(* Logix 5000 AddOnInstructionDefinition export NORD_ADC; software revision 24.02; part 2 of 3 *)
(* tags used below, declared in another part *)
   ParameterNumber : INT;
   ParameterIndex : SINT;
   ParameterSet : SINT;
   Done : BOOL;
   Busy : BOOL;
   ReadMsg : MESSAGE;   // Read Msg to Module
   ReadTrigger : BOOL;
   ReadValue : DINT;   // Read Value from message
   WriteMsg : MESSAGE;   // Write Msg to Module
   WriteTrigger : BOOL;
   WriteValue : DINT;
   Error : BOOL;
   VFD_NotPresent : BOOL;   // VFD not present in Localbus
   EthernetDisconnected : BOOL;   // Eth. cord to Module is disconnected
   Backup : NORD_ParameterBackup;   // Parameter Backup File
   CompletionPercent : DINT;   // Backup/Restore Complete Percentage
   GetID_InProcess : BOOL;
   BackupInProcess : BOOL;
   RestoreInProcess : BOOL;
   HasInternalPLC : BOOL;
   ErrorID : DINT;   // Message Error Code
   WriteValueMSG : DINT;
   Instance : INT;
   HasParamIndex : BOOL;   // Set Parameter has Indexes
   HasParamSets : BOOL;   // Set Parameter has Parameter Sets
   ReadErrorOS : BOOL;
   WriteErrorONS : BOOL;
   TrigONS1 : BOOL;
   ReadDoneOS : BOOL;
   WriteDoneONS : BOOL;
   MacAddr : SINT[6];   // MAC Address of CU/TU
   GetID_ReadTrigger : BOOL;
   BackupSM : INT;   // 0: Not Active 10: Reset indexes 20: Clear Old Backup 30: Reset Indexes 40: Prepare Read Msg 50: Read Trigger 60: Read Co
   Index : INT;
   DeviceID : STRING;   // Device ID of VFD
   RestoreSM : INT;   // 0: Not Active 10: Reset Indexes 15: # of Saved Param 20: Get RestoreParam 21: Prepare Read Msg 22: Read Trigger 23: Read
   Index1 : INT;   // Store Index: VFD
   IndexInst : INT;   // Instance Index
   RestoreParam : INT;   // Parameter Number to be Restored
   SavedParamsVFD : INT;
   BackupReadTrigger : BOOL;
   RestWriteTrig : BOOL;
   RestIndexONS : BOOL;
   RestReadTrig : BOOL;
   BackupLast : BOOL;   // Determines Backup/Restore Complete Percentage Calculation
   WriteSM : SINT;   // 0: Not Active 10: Write LEN=4 20: 1st WriteTrigger 30: Write Complete - 40: Write LEN=2 - 50: 2nd WriteTrigger 60: Write
   Class : INT;
   TrigONS2 : BOOL;
   NumOfParams : DINT;   // Number of parameters in the VFD
   WriteTriggerONS : BOOL;
   WriteTrigInternal : BOOL;   // 1st Attempt: LEN = 4 2nd Attempt: LEN = 2
   Write16Bit : BOOL;   // 0: Write LEN=4 1: Write LEN=2
   AOI_FirstScan : BOOL;   // First Scan of AOI
   Percent100ONS : BOOL;
   GetID_Done_ONS : BOOL;
   Index2 : INT;   // Store Index: CU/TU
   SavedParamsCTU : INT;
   RestoreCTU : BOOL;   // Restore CTU Parameters
   RestIndexONS2 : BOOL;
   CompPercentIndex : INT;
   StoreDevID : BOOL;
   StoreDevID_DN : BOOL;
   ResetIndexes : BOOL;
   ResetIndexDN : BOOL;
   GetRestParam : BOOL;   // Get Restore Parameter Logic
   GetRestParamDN : BOOL;   // Got Restore Param
   ResetMsgEr : BOOL;
   RestoreFailed : BOOL;   // All writes in restore failed
   RestoreFailedONS : BOOL;
   RestoreHasWrite : BOOL;
   RestoreHasWriteONS : BOOL;
(* NORD_ADC, continued *)

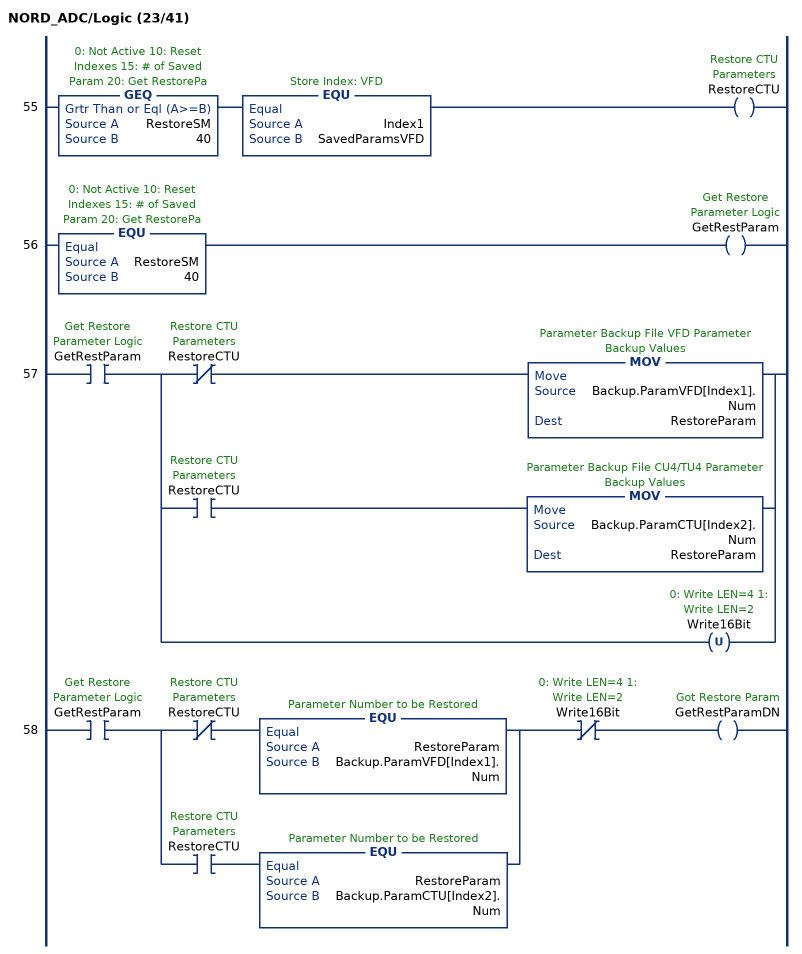
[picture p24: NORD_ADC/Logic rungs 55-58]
   55: GEQ(RestoreSM,40)EQU(Index1,SavedParamsVFD)OTE(RestoreCTU);
   56: EQU(RestoreSM,40)OTE(GetRestParam);
   57: XIC(GetRestParam)[XIO(RestoreCTU) MOV(Backup.ParamVFD[Index1].Num,RestoreParam) ,XIC(RestoreCTU) MOV(Backup.ParamCTU[Index2].Num,RestoreParam) ,OTU(Write16Bit) ];
   58: XIC(GetRestParam)[XIO(RestoreCTU) EQU(RestoreParam,Backup.ParamVFD[Index1].Num) ,XIC(RestoreCTU) EQU(RestoreParam,Backup.ParamCTU[Index2].Num) ]XIO(Write16Bit)OTE(GetRestParamDN);
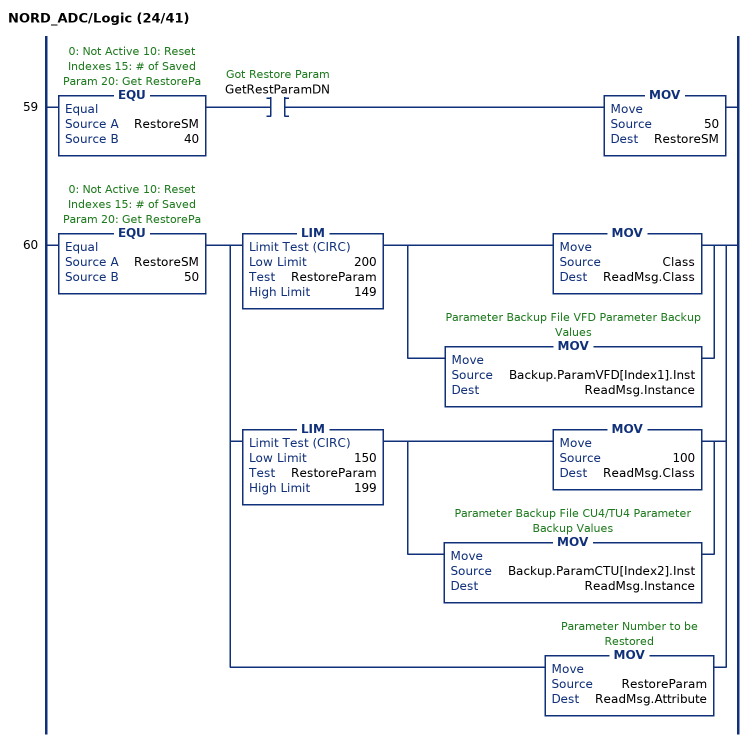
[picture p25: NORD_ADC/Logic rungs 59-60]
   59: EQU(RestoreSM,40)XIC(GetRestParamDN)MOV(50,RestoreSM);
   60: EQU(RestoreSM,50)[[LIM(200,RestoreParam,149) [MOV(Class,ReadMsg.Class) ,MOV(Backup.ParamVFD[Index1].Inst,ReadMsg.Instance) ] ,LIM(150,RestoreParam,199) [MOV(100,ReadMsg.Class) ,MOV(Backup.ParamCTU[Index2].Inst,ReadMsg.Instance) ] ] ,MOV(RestoreParam,ReadMsg.Attribute) ];
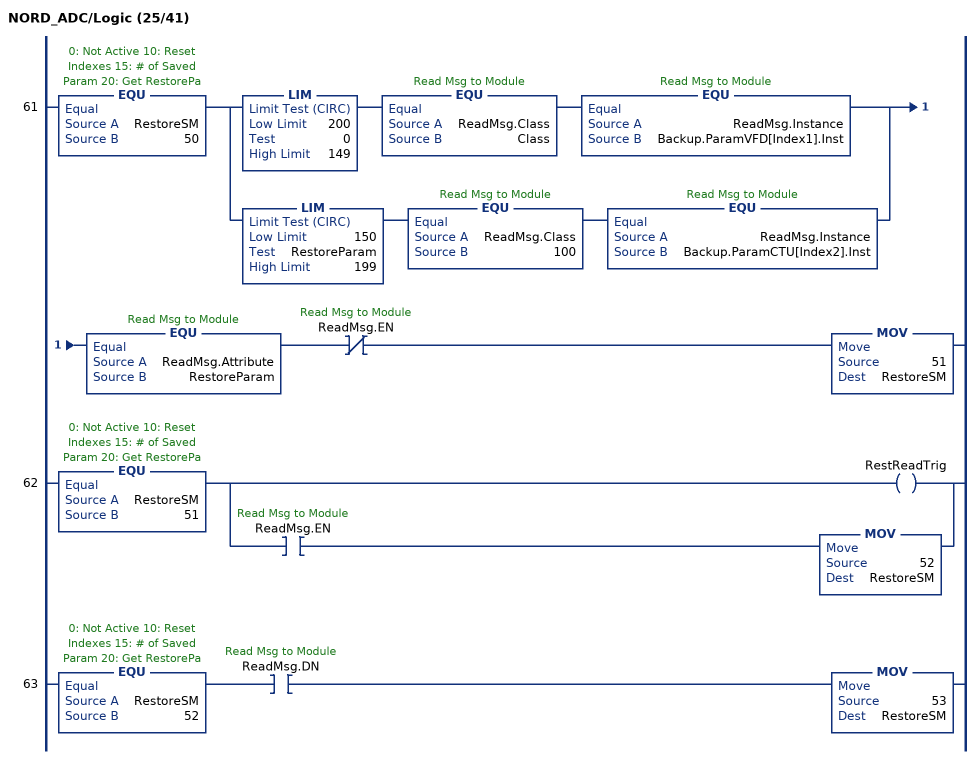
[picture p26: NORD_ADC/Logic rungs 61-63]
   61: EQU(RestoreSM,50)[LIM(200,0,149) EQU(ReadMsg.Class,Class) EQU(ReadMsg.Instance,Backup.ParamVFD[Index1].Inst) ,LIM(150,RestoreParam,199) EQU(ReadMsg.Class,100) EQU(ReadMsg.Instance,Backup.ParamCTU[Index2].Inst) ]EQU(ReadMsg.Attribute,RestoreParam)XIO(ReadMsg.EN)MOV(51,RestoreSM);
   62: EQU(RestoreSM,51)[OTE(RestReadTrig) ,XIC(ReadMsg.EN) MOV(52,RestoreSM) ];
   63: EQU(RestoreSM,52)XIC(ReadMsg.DN)MOV(53,RestoreSM);
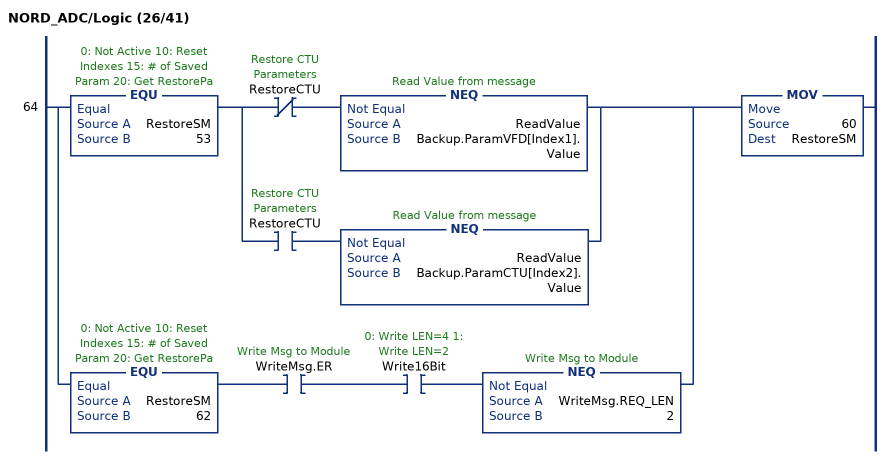
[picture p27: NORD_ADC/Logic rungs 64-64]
   64: [EQU(RestoreSM,53) [XIO(RestoreCTU) NEQ(ReadValue,Backup.ParamVFD[Index1].Value) ,XIC(RestoreCTU) NEQ(ReadValue,Backup.ParamCTU[Index2].Value) ] ,EQU(RestoreSM,62) XIC(WriteMsg.ER) XIC(Write16Bit) NEQ(WriteMsg.REQ_LEN,2) ]MOV(60,RestoreSM);
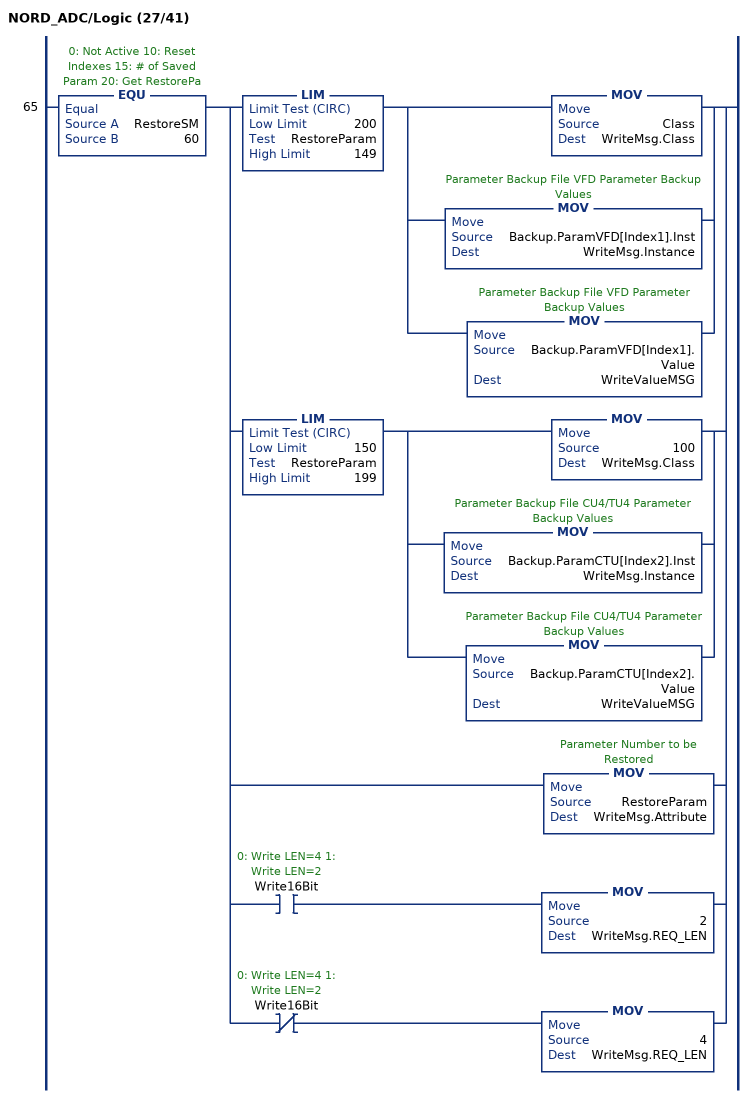
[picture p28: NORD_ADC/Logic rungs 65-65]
   65: EQU(RestoreSM,60)[[LIM(200,RestoreParam,149) [MOV(Class,WriteMsg.Class) ,[MOV(Backup.ParamVFD[Index1].Inst,WriteMsg.Instance) ,MOV(Backup.ParamVFD[Index1].Value,WriteValueMSG) ] ] ,LIM(150,RestoreParam,199) [MOV(100,WriteMsg.Class) ,MOV(Backup.ParamCTU[Index2].Inst,WriteMsg.Instance) ,MOV(Backup.ParamCTU[Index2].Value,WriteValueMSG) ] ] ,MOV(RestoreParam,WriteMsg.Attribute) ,XIC(Write16Bit) MOV(2,WriteMsg.REQ_LEN) ,XIO(Write16Bit) MOV(4,WriteMsg.REQ_LEN) ];
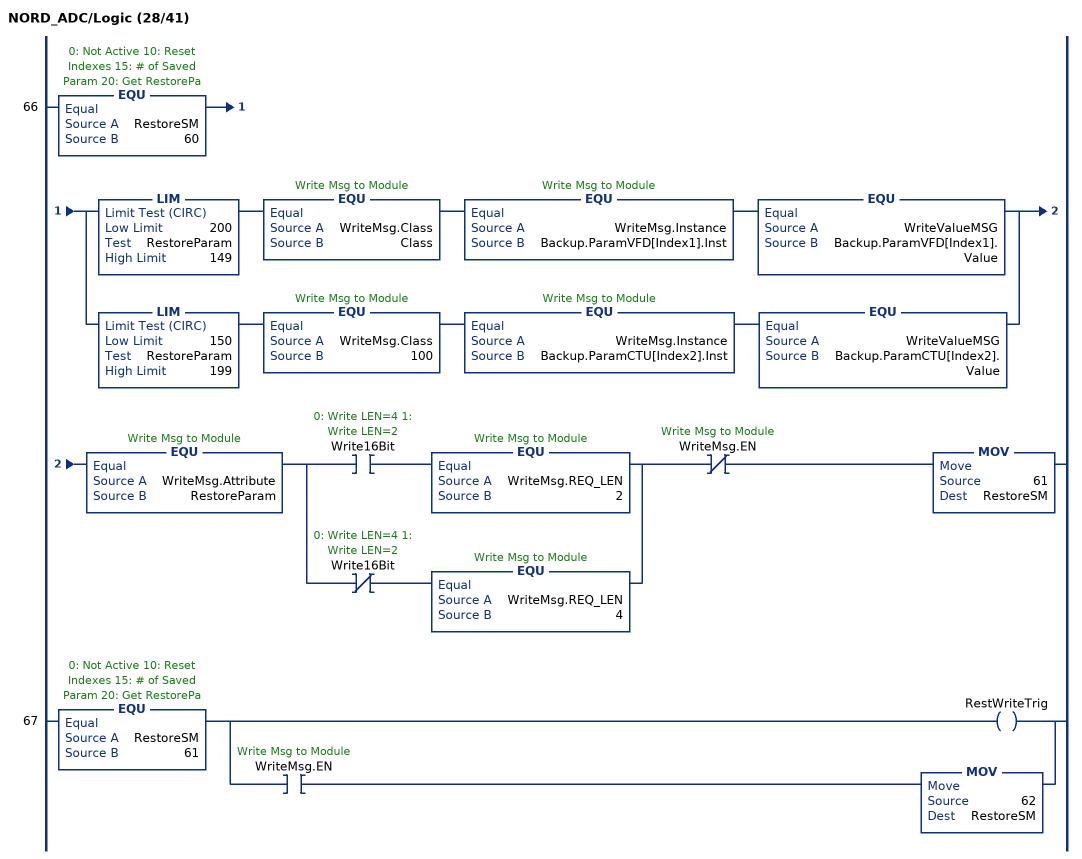
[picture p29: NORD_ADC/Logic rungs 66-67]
   66: EQU(RestoreSM,60)[LIM(200,RestoreParam,149) EQU(WriteMsg.Class,Class) EQU(WriteMsg.Instance,Backup.ParamVFD[Index1].Inst) EQU(WriteValueMSG,Backup.ParamVFD[Index1].Value) ,LIM(150,RestoreParam,199) EQU(WriteMsg.Class,100) EQU(WriteMsg.Instance,Backup.ParamCTU[Index2].Inst) EQU(WriteValueMSG,Backup.ParamCTU[Index2].Value) ]EQU(WriteMsg.Attribute,RestoreParam)[XIC(Write16Bit) EQU(WriteMsg.REQ_LEN,2) ,XIO(Write16Bit) EQU(WriteMsg.REQ_LEN,4) ]XIO(WriteMsg.EN)MOV(61,RestoreSM);
   67: EQU(RestoreSM,61)[OTE(RestWriteTrig) ,XIC(WriteMsg.EN) MOV(62,RestoreSM) ];
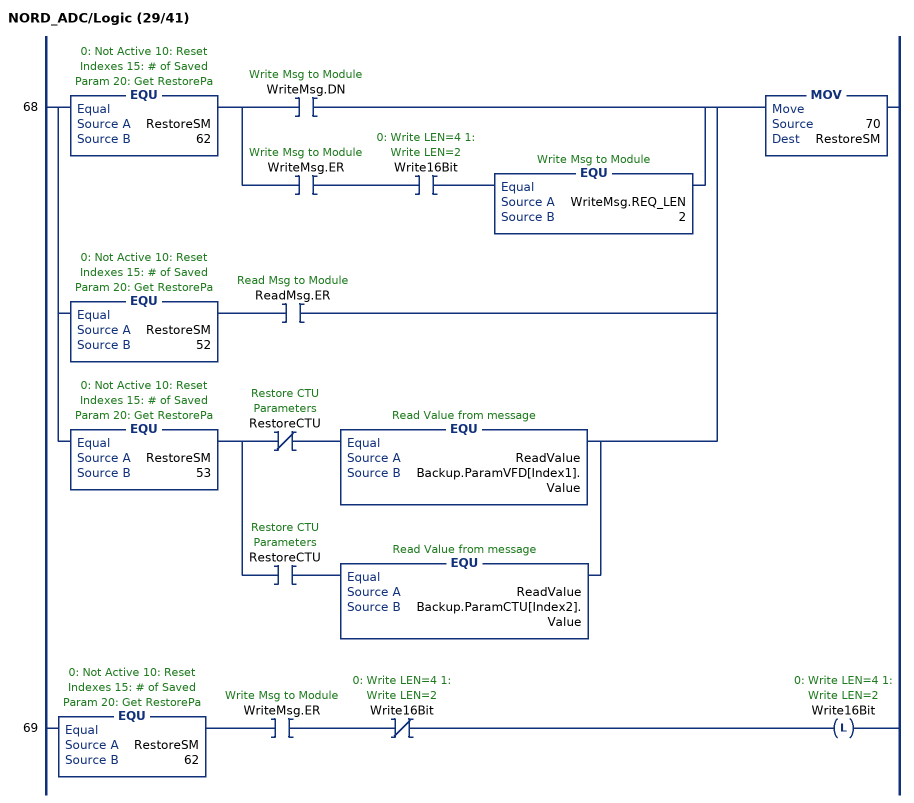
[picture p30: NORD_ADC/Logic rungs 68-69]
   68: [EQU(RestoreSM,62) [XIC(WriteMsg.DN) ,XIC(WriteMsg.ER) XIC(Write16Bit) EQU(WriteMsg.REQ_LEN,2) ] ,EQU(RestoreSM,52) XIC(ReadMsg.ER) ,EQU(RestoreSM,53) [XIO(RestoreCTU) EQU(ReadValue,Backup.ParamVFD[Index1].Value) ,XIC(RestoreCTU) EQU(ReadValue,Backup.ParamCTU[Index2].Value) ] ]MOV(70,RestoreSM);
   69: EQU(RestoreSM,62)XIC(WriteMsg.ER)XIO(Write16Bit)OTL(Write16Bit);
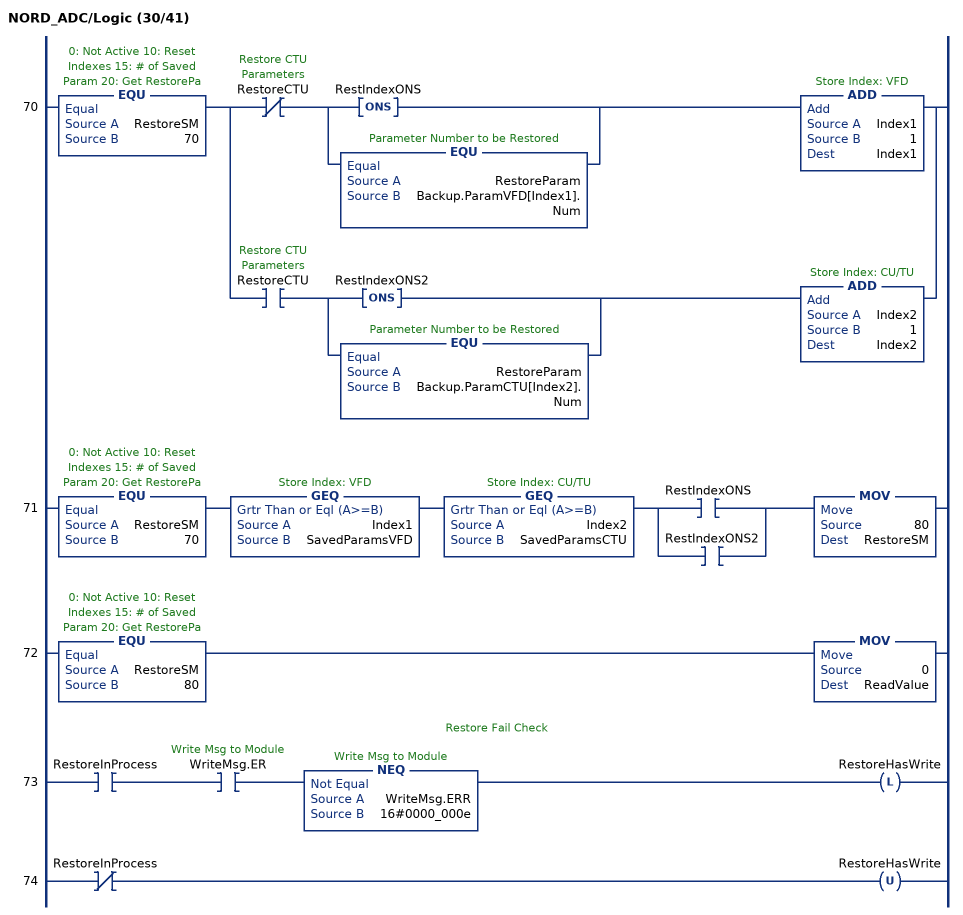
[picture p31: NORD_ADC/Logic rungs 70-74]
   70: EQU(RestoreSM,70)[XIO(RestoreCTU) [ONS(RestIndexONS) ,EQU(RestoreParam,Backup.ParamVFD[Index1].Num) ] ADD(Index1,1,Index1) ,XIC(RestoreCTU) [ONS(RestIndexONS2) ,EQU(RestoreParam,Backup.ParamCTU[Index2].Num) ] ADD(Index2,1,Index2) ];
   71: EQU(RestoreSM,70)GEQ(Index1,SavedParamsVFD)GEQ(Index2,SavedParamsCTU)[XIC(RestIndexONS) ,XIC(RestIndexONS2) ]MOV(80,RestoreSM);
   72: EQU(RestoreSM,80)MOV(0,ReadValue);
   // Restore Fail Check
   73: XIC(RestoreInProcess)XIC(WriteMsg.ER)NEQ(WriteMsg.ERR,16#0000_000e)OTL(RestoreHasWrite);
   74: XIO(RestoreInProcess)OTU(RestoreHasWrite);
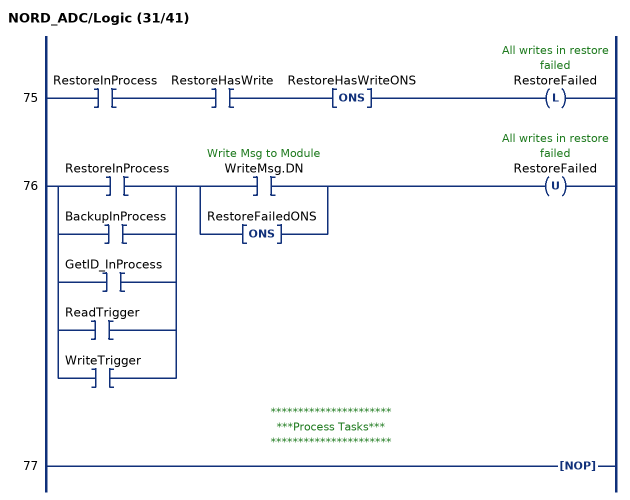
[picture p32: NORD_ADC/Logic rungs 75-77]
   75: XIC(RestoreInProcess)XIC(RestoreHasWrite)ONS(RestoreHasWriteONS)OTL(RestoreFailed);
   76: [XIC(RestoreInProcess) ,XIC(BackupInProcess) ,XIC(GetID_InProcess) ,XIC(ReadTrigger) ,XIC(WriteTrigger) ][XIC(WriteMsg.DN) ,ONS(RestoreFailedONS) ]OTU(RestoreFailed);
   // **********************
   // ***Process Tasks***
   // **********************
   77: NOP();
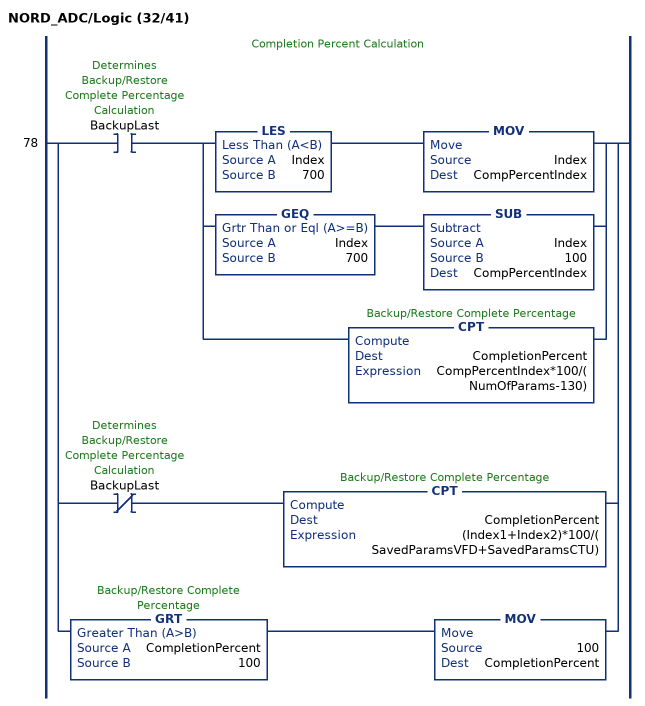
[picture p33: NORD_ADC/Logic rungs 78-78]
   // Completion Percent Calculation
   78: [XIC(BackupLast) [[LES(Index,700) MOV(Index,CompPercentIndex) ,GEQ(Index,700) SUB(Index,100,CompPercentIndex) ] ,CPT(CompletionPercent,CompPercentIndex*100/(NumOfParams-130)) ] ,XIO(BackupLast) CPT(CompletionPercent,(Index1+Index2)*100/(SavedParamsVFD+SavedParamsCTU)) ,GRT(CompletionPercent,100) MOV(100,CompletionPercent) ];
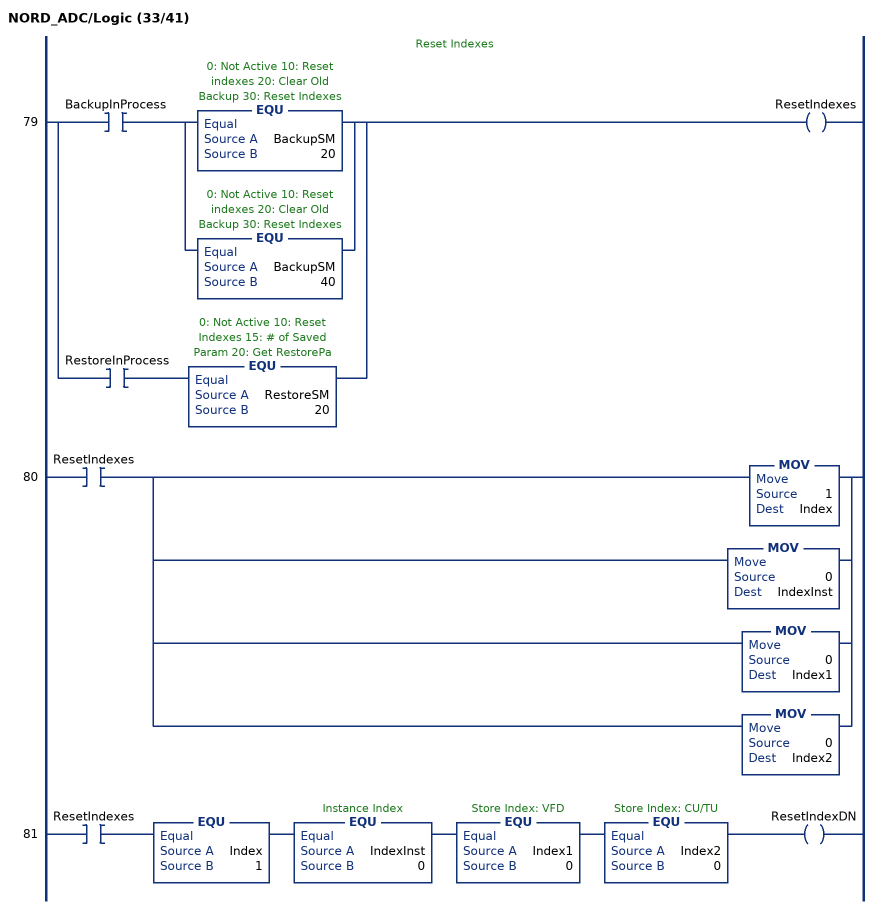
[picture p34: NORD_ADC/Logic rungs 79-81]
   // Reset Indexes
   79: [XIC(BackupInProcess) [EQU(BackupSM,20) ,EQU(BackupSM,40) ] ,XIC(RestoreInProcess) EQU(RestoreSM,20) ]OTE(ResetIndexes);
   80: XIC(ResetIndexes)[MOV(1,Index) ,MOV(0,IndexInst) ,MOV(0,Index1) ,MOV(0,Index2) ];
   81: XIC(ResetIndexes)EQU(Index,1)EQU(IndexInst,0)EQU(Index1,0)EQU(Index2,0)OTE(ResetIndexDN);
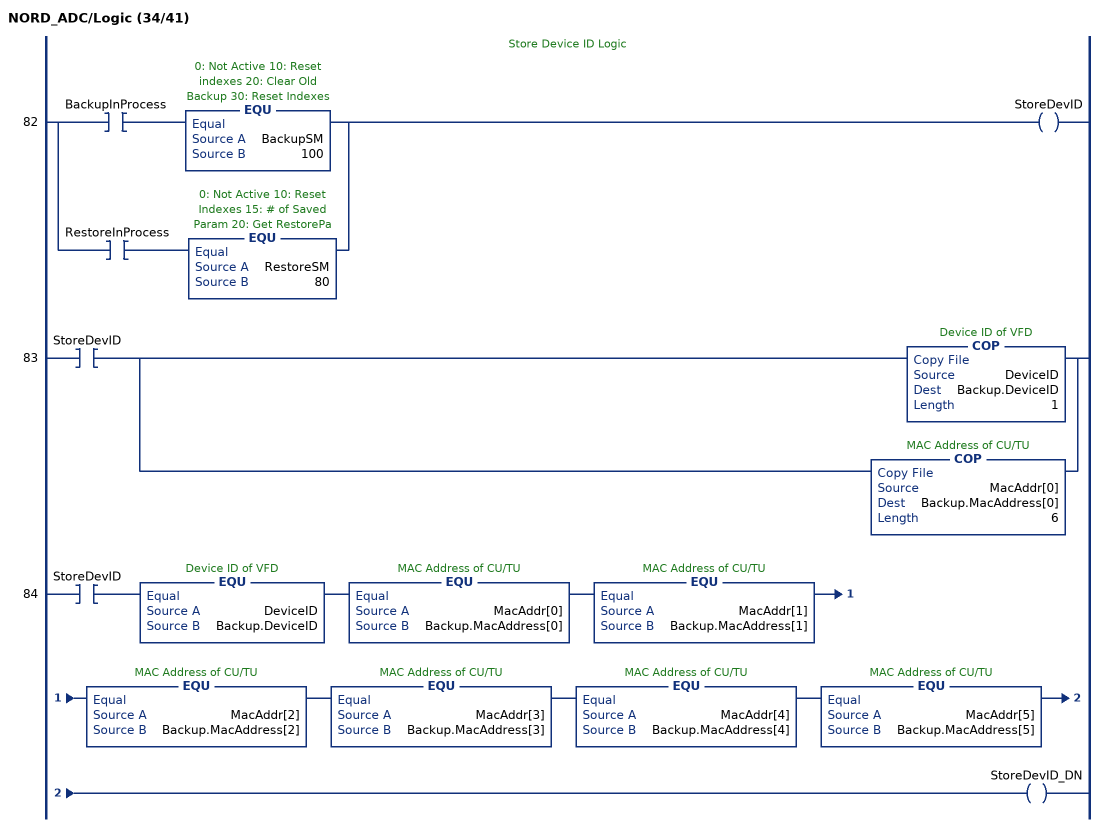
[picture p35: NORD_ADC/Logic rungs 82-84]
   // Store Device ID Logic
   82: [XIC(BackupInProcess) EQU(BackupSM,100) ,XIC(RestoreInProcess) EQU(RestoreSM,80) ]OTE(StoreDevID);
   83: XIC(StoreDevID)[COP(DeviceID,Backup.DeviceID,1) ,COP(MacAddr[0],Backup.MacAddress[0],6) ];
   84: XIC(StoreDevID)EQU(DeviceID,Backup.DeviceID)EQU(MacAddr[0],Backup.MacAddress[0])EQU(MacAddr[1],Backup.MacAddress[1])EQU(MacAddr[2],Backup.MacAddress[2])EQU(MacAddr[3],Backup.MacAddress[3])EQU(MacAddr[4],Backup.MacAddress[4])EQU(MacAddr[5],Backup.MacAddress[5])OTE(StoreDevID_DN);
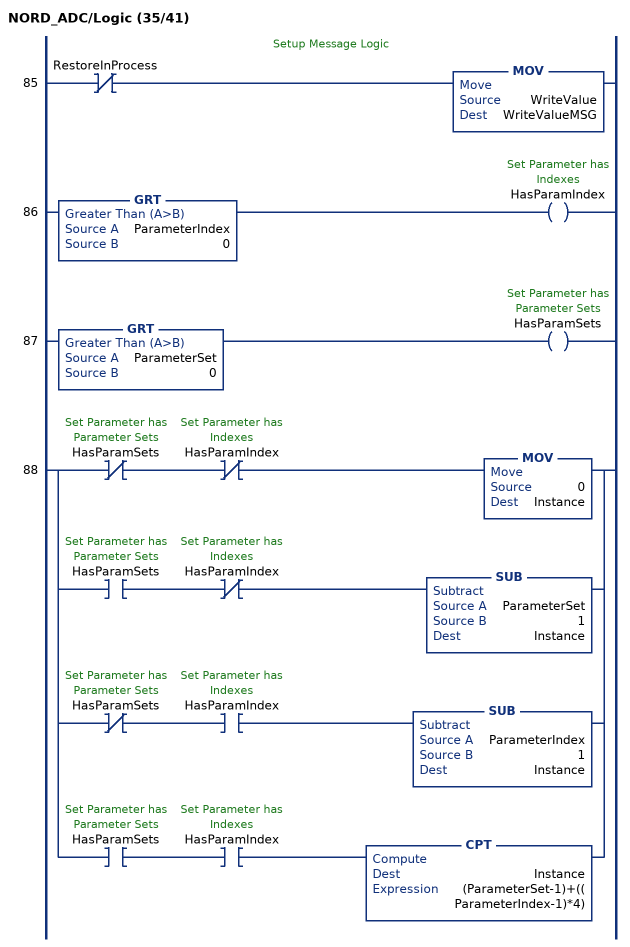
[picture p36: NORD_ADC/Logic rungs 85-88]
   // Setup Message Logic
   85: XIO(RestoreInProcess)MOV(WriteValue,WriteValueMSG);
   86: GRT(ParameterIndex,0)OTE(HasParamIndex);
   87: GRT(ParameterSet,0)OTE(HasParamSets);
   88: [XIO(HasParamSets) XIO(HasParamIndex) MOV(0,Instance) ,XIC(HasParamSets) XIO(HasParamIndex) SUB(ParameterSet,1,Instance) ,XIO(HasParamSets) XIC(HasParamIndex) SUB(ParameterIndex,1,Instance) ,XIC(HasParamSets) XIC(HasParamIndex) CPT(Instance,(ParameterSet-1)+((ParameterIndex-1)*4)) ];
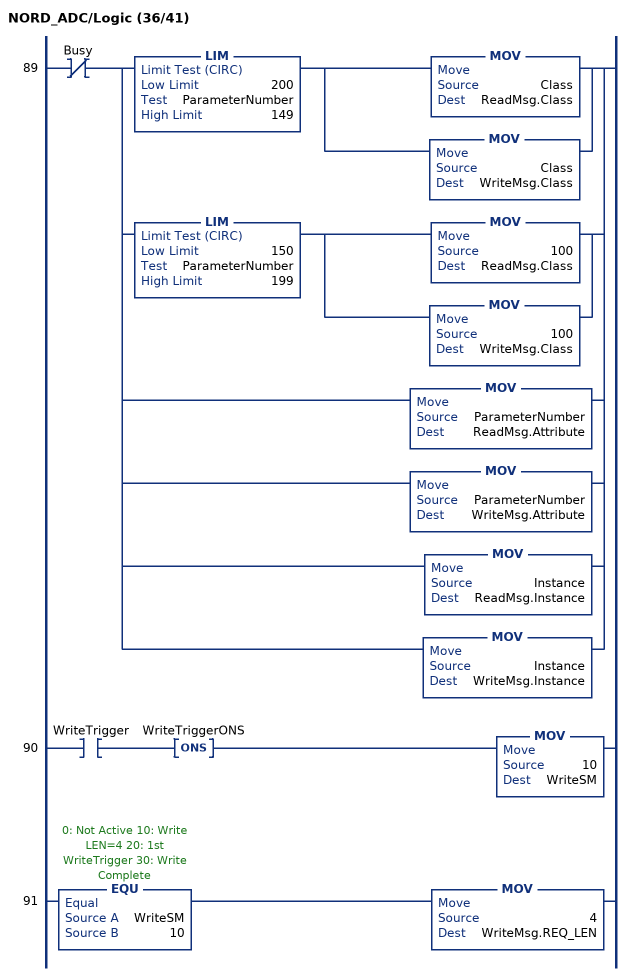
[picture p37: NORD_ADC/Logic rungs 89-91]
   89: XIO(Busy)[[LIM(200,ParameterNumber,149) [MOV(Class,ReadMsg.Class) ,MOV(Class,WriteMsg.Class) ] ,LIM(150,ParameterNumber,199) [MOV(100,ReadMsg.Class) ,MOV(100,WriteMsg.Class) ] ] ,[MOV(ParameterNumber,ReadMsg.Attribute) ,MOV(ParameterNumber,WriteMsg.Attribute) ] ,[MOV(Instance,ReadMsg.Instance) ,MOV(Instance,WriteMsg.Instance) ] ];
   90: XIC(WriteTrigger)ONS(WriteTriggerONS)MOV(10,WriteSM);
   91: EQU(WriteSM,10)MOV(4,WriteMsg.REQ_LEN);
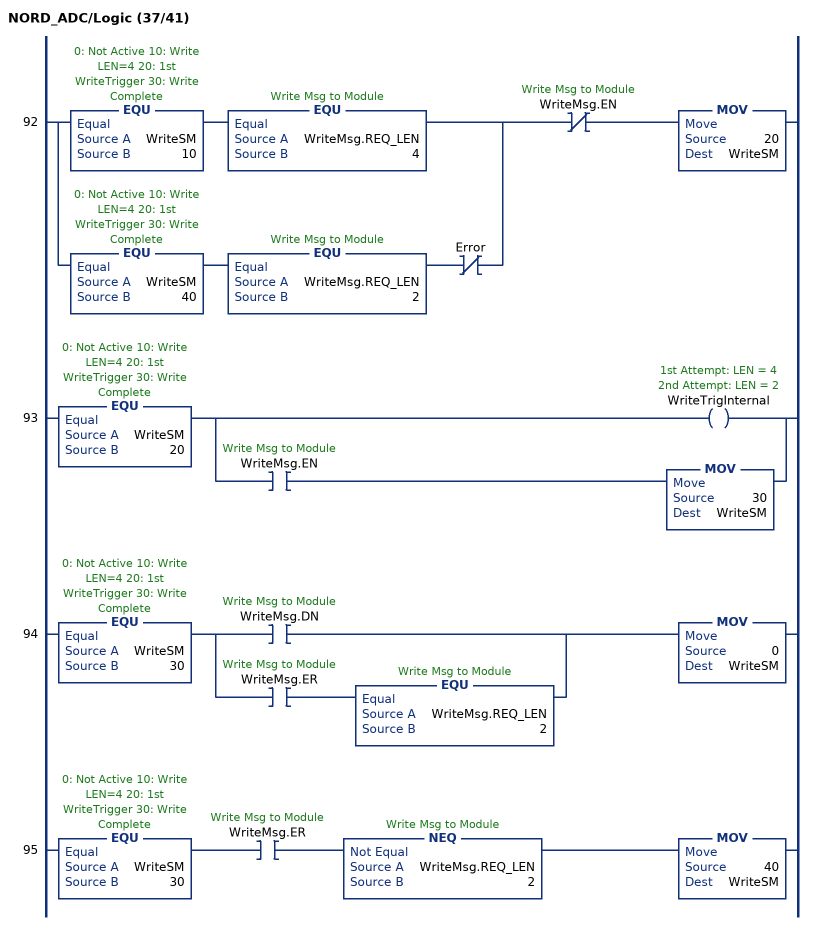
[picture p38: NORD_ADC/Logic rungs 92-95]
   92: [EQU(WriteSM,10) EQU(WriteMsg.REQ_LEN,4) ,EQU(WriteSM,40) EQU(WriteMsg.REQ_LEN,2) XIO(Error) ]XIO(WriteMsg.EN)MOV(20,WriteSM);
   93: EQU(WriteSM,20)[OTE(WriteTrigInternal) ,XIC(WriteMsg.EN) MOV(30,WriteSM) ];
   94: EQU(WriteSM,30)[XIC(WriteMsg.DN) ,XIC(WriteMsg.ER) EQU(WriteMsg.REQ_LEN,2) ]MOV(0,WriteSM);
   95: EQU(WriteSM,30)XIC(WriteMsg.ER)NEQ(WriteMsg.REQ_LEN,2)MOV(40,WriteSM);
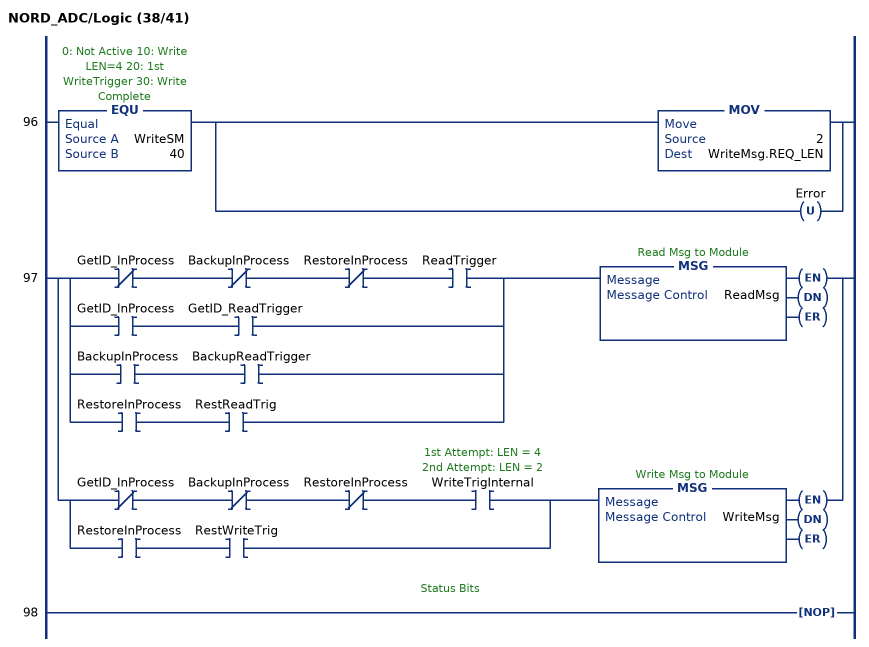
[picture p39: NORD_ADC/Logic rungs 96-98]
   96: EQU(WriteSM,40)[MOV(2,WriteMsg.REQ_LEN) ,OTU(Error) ];
   97: [[XIO(GetID_InProcess) XIO(BackupInProcess) XIO(RestoreInProcess) XIC(ReadTrigger) ,XIC(GetID_InProcess) XIC(GetID_ReadTrigger) ,XIC(BackupInProcess) XIC(BackupReadTrigger) ,XIC(RestoreInProcess) XIC(RestReadTrig) ] MSG(ReadMsg) ,[XIO(GetID_InProcess) XIO(BackupInProcess) XIO(RestoreInProcess) XIC(WriteTrigInternal) ,XIC(RestoreInProcess) XIC(RestWriteTrig) ] MSG(WriteMsg) ];
   // Status Bits
   98: NOP();
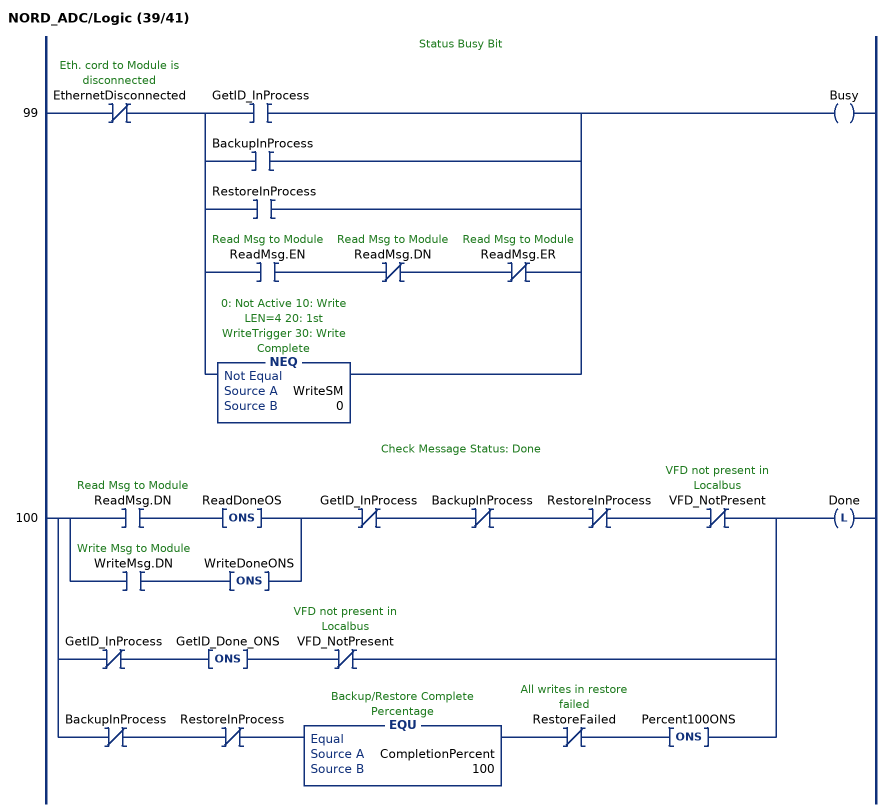
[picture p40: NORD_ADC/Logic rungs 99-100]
   // Status Busy Bit
   99: XIO(EthernetDisconnected)[XIC(GetID_InProcess) ,XIC(BackupInProcess) ,XIC(RestoreInProcess) ,XIC(ReadMsg.EN) XIO(ReadMsg.DN) XIO(ReadMsg.ER) ,NEQ(WriteSM,0) ]OTE(Busy);
   // Check Message Status: Done
   100: [[XIC(ReadMsg.DN) ONS(ReadDoneOS) ,XIC(WriteMsg.DN) ONS(WriteDoneONS) ] XIO(GetID_InProcess) XIO(BackupInProcess) XIO(RestoreInProcess) XIO(VFD_NotPresent) ,XIO(GetID_InProcess) ONS(GetID_Done_ONS) XIO(VFD_NotPresent) ,XIO(BackupInProcess) XIO(RestoreInProcess) EQU(CompletionPercent,100) XIO(RestoreFailed) ONS(Percent100ONS) ]OTL(Done);
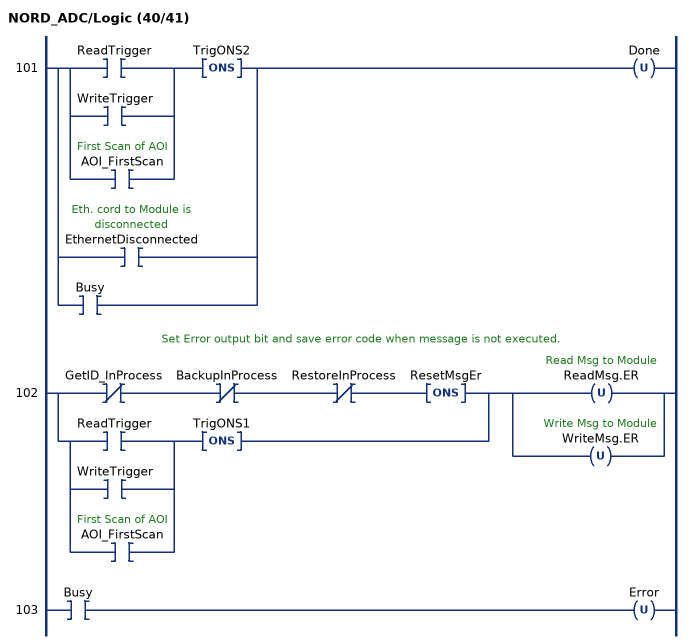
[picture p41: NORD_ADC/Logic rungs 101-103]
   101: [[XIC(ReadTrigger) ,XIC(WriteTrigger) ,XIC(AOI_FirstScan) ] ONS(TrigONS2) ,XIC(EthernetDisconnected) ,XIC(Busy) ]OTU(Done);
   // Set Error output bit and save error code when message is not executed.
   102: [XIO(GetID_InProcess) XIO(BackupInProcess) XIO(RestoreInProcess) ONS(ResetMsgEr) ,[XIC(ReadTrigger) ,XIC(WriteTrigger) ,XIC(AOI_FirstScan) ] ONS(TrigONS1) ][OTU(ReadMsg.ER) ,OTU(WriteMsg.ER) ];
   103: XIC(Busy)OTU(Error);
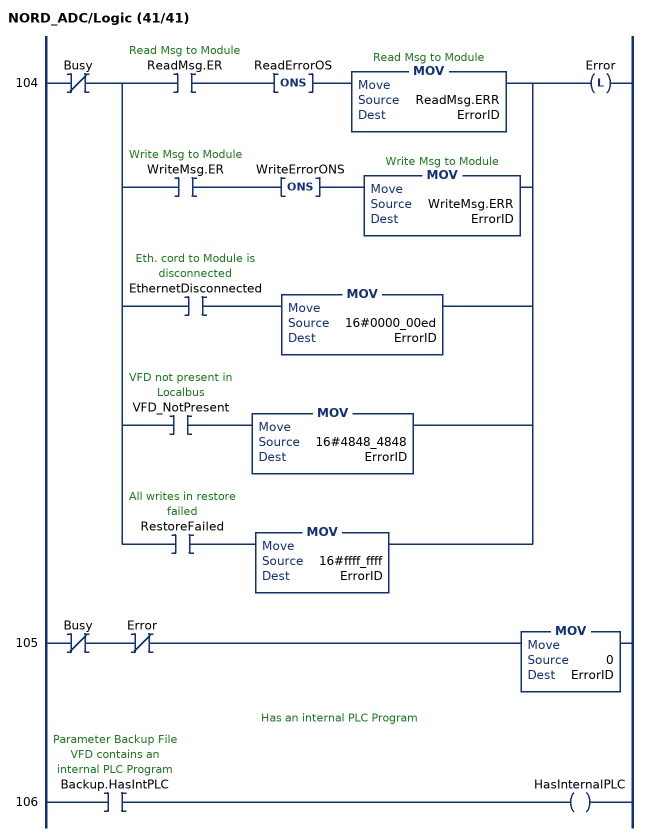
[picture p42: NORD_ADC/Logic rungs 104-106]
   104: XIO(Busy)[XIC(ReadMsg.ER) ONS(ReadErrorOS) MOV(ReadMsg.ERR,ErrorID) ,XIC(WriteMsg.ER) ONS(WriteErrorONS) MOV(WriteMsg.ERR,ErrorID) ,XIC(EthernetDisconnected) MOV(16#0000_00ed,ErrorID) ,XIC(VFD_NotPresent) MOV(16#4848_4848,ErrorID) ,XIC(RestoreFailed) MOV(16#ffff_ffff,ErrorID) ]OTL(Error);
   105: XIO(Busy)XIO(Error)MOV(0,ErrorID);
   // Has an internal PLC Program
   106: XIC(Backup.HasIntPLC)OTE(HasInternalPLC);
END_ROUTINE
